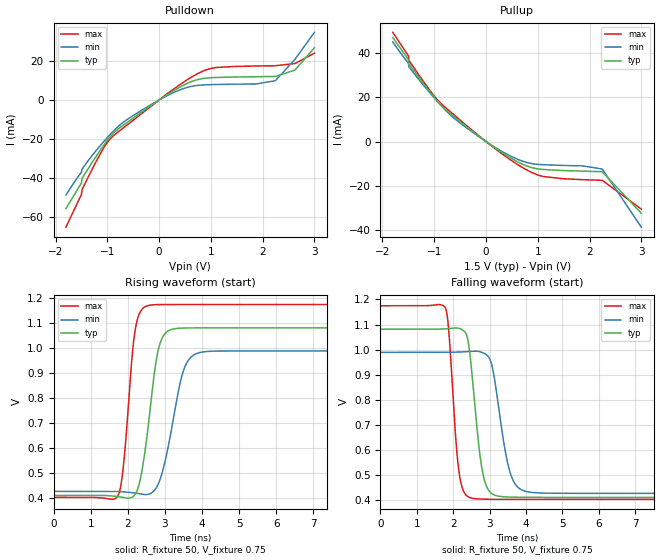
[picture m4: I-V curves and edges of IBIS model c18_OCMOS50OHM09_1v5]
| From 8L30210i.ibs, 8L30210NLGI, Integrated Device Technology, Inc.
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| 3.25758e+00   -6.92224e-03   -1.23527e+00   -1.07149e-03
| 3.33333e+00   -4.29506e-02   -2.23637e+00   -4.11997e-03
| 3.40909e+00   -5.86135e-01   -3.23815e+00   -1.02974e-02
| 3.48485e+00   -1.79017e+00   -4.24043e+00   -2.01278e-02
| 3.56061e+00   -2.99495e+00   -5.24309e+00   -7.87092e-02
| 3.63636e+00   -4.20024e+00   -6.24602e+00   -1.11369e+00
| 3.71212e+00   -5.40590e+00   -7.24916e+00   -2.65555e+00
| 3.78788e+00   -6.61182e+00   -8.25246e+00   -4.19783e+00
| 3.86364e+00   -7.81792e+00   -9.25587e+00   -5.74035e+00
| 3.93939e+00   -9.02412e+00   -1.02594e+01   -7.28299e+00
| 4.01515e+00   -1.02304e+01   -1.12629e+01   -8.82567e+00
| 4.09091e+00   -1.14366e+01   -1.22664e+01   -1.03683e+01
| 4.16667e+00   -1.26429e+01   -1.32700e+01   -1.19109e+01
| 4.24242e+00   -1.38491e+01   -1.42735e+01   -1.34534e+01
| 4.31818e+00   -1.50552e+01   -1.52769e+01   -1.49957e+01
| 4.39394e+00   -1.62613e+01   -1.62803e+01   -1.65379e+01
| 4.46970e+00   -1.74672e+01   -1.72837e+01   -1.80799e+01
| 4.54545e+00   -1.86730e+01   -1.82870e+01   -1.96217e+01
| 4.62121e+00   -1.98787e+01   -1.92902e+01   -2.11633e+01
| 4.69697e+00   -2.10843e+01   -2.02933e+01   -2.27047e+01
| 4.77273e+00   -2.22897e+01   -2.12963e+01   -2.42459e+01
| 4.84848e+00   -2.34950e+01   -2.22993e+01   -2.57868e+01
| 4.92424e+00   -2.47001e+01   -2.33021e+01   -2.73276e+01
| 5.00000e+00   -2.59051e+01   -2.43049e+01   -2.88681e+01
[Model] c18_OCMOS50OHM09_1v5
Model_type   Output
Polarity   Non-Inverting
|   typ   min   max
C_comp   2pF   1.5pF   2.5pF
Vmeas = .75
Rref = 50
Cref = 0
Vref = .75
|   typ   min   max
[Voltage range]   1.5V   1.4V   1.6V
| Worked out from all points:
|   slope of the pulldown table from 0 to 0.225 V, typ, clamps not added: 57.6 ohm
|   slope of the pullup table from 0 to 0.225 V, typ, clamps not added: 60.7 ohm
|   rising waveform, R_fixture 50, V_fixture 0.75: 20-80 % time 340ps typ, 442ps min, 249ps max; typ from 0.411 V to 1.08 V
|   falling waveform, R_fixture 50, V_fixture 0.75: 20-80 % time 282ps typ, 367ps min, 216ps max; typ from 1.08 V to 0.411 V
[Pulldown]
|Voltage   I (typ)   I (min)   I (max)
-1.8V     -55.9mA    -48.94mA   -65.46mA
-1.5V     -42.72mA   -37.09mA   -48.61mA
-1.49V    -40.39mA   -35.66mA   -46.16mA
-1.46V    -39.13mA   -34.53mA   -44.55mA
-983.9mV  -20.19mA   -18.82mA   -21.25mA
-596.9mV  -11.15mA   -9.665mA   -12.41mA
355.7mV   5.967mA    4.71mA     7.053mA
683.2mV   10.01mA    7.301mA    12.66mA
1.011V    11.47mA    7.909mA    16.3mA
2.244V    12.1mA     9.921mA    17.62mA
2.622V    15.39mA    20.88mA    18.75mA
3V        26.87mA    34.82mA    24.1mA
[Pullup]
|Voltage   I (typ)   I (min)   I (max)
-1.8V     46.88mA    44.9mA     49.25mA
-1.5V     37.02mA    35.28mA    38.64mA
-1.49V    35.08mA    33.75mA    36.58mA
-924.4mV  17.94mA    17.66mA    18.44mA
-686.2mV  12.56mA    11.93mA    13.37mA
-477.8mV  8.614mA    7.966mA    9.22mA
385.5mV   -6.144mA   -5.463mA   -6.836mA
772.5mV   -10.87mA   -9.341mA   -12.62mA
1.1V      -12.58mA   -10.44mA   -15.72mA
1.866V    -13.36mA   -10.98mA   -17.19mA
2.244V    -13.6mA    -12.37mA   -17.48mA
3V        -32.35mA   -38.61mA   -30.46mA
[Ramp]
|   typ   min   max
dV/dt_r   0.408/0.347n   0.344/0.454n   0.467/0.252n
dV/dt_f   0.405/0.283n   0.339/0.369n   0.465/0.217n
R_load =   50.0000
[Rising Waveform]
R_fixture = 50
V_fixture = 0.75   |Vcc_typ
V_fixture_min = 0.70 |Vcc_min
V_fixture_max = 0.80 |Vcc_max
C_fixture = 0.0p
| Time   typ   min   max
0s        411.1mV    427.1mV    403.3mV
1.74ns    406.3mV    426.5mV    412.3mV
1.892ns   402.4mV    425mV      544.2mV
2.178ns   411.7mV    421mV      1.052V
2.463ns   587.4mV    414.3mV    1.165V
2.739ns   925.8mV    435.2mV    1.174V
2.9ns     1.032V     488.9mV    1.174V
3.452ns   1.08V      887.3mV    1.175V
3.794ns   1.081V     974.3mV    1.175V
9.49ns    1.081V     989mV      1.175V
[Falling Waveform]
R_fixture = 50
V_fixture = 0.75   |Vcc_typ
V_fixture_min = 0.70  |Vcc_min
V_fixture_max = 0.80  |Vcc_max
C_fixture = 0.0p
| Time   typ   min   max
0s        1.081V     989mV      1.175V
1.788ns   1.083V     988.9mV    1.165V
1.883ns   1.084V     989.1mV    1.068V
2.14ns    1.085V     990.1mV    536mV
2.415ns   1.029V     992.2mV    413.2mV
2.777ns   537.7mV    989.8mV    404.2mV
3.081ns   424.2mV    926.6mV    403.5mV
3.509ns   412.4mV    540.3mV    403.3mV
3.87ns    411.3mV    441.9mV    403.3mV
9.49ns    411.1mV    427.1mV    403.3mV
